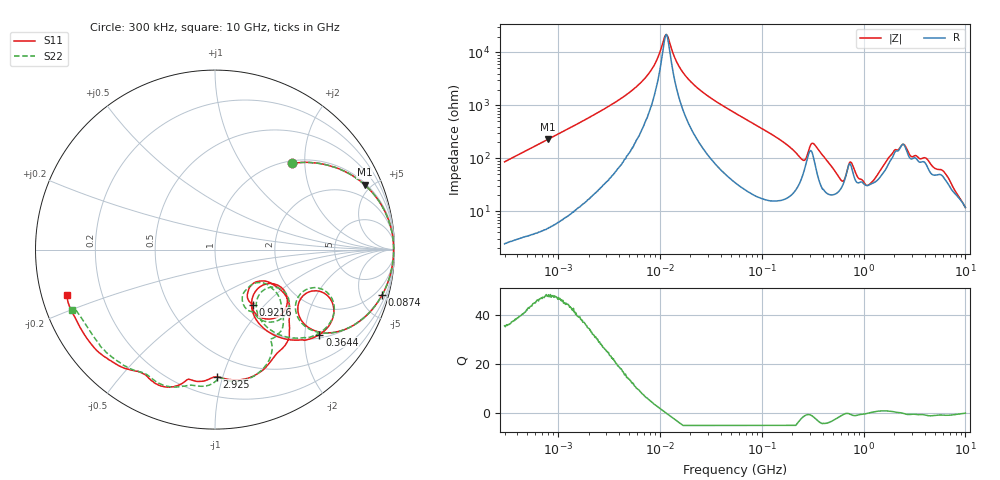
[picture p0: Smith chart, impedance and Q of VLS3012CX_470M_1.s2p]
! S-Parameter Data Generated by TDK Corporation
! Copyright(C) 2019 TDK Corporation.
! All Rights Reserved.
! TDK P/N: VLS3012CX-470M-1 (Inductor)
! Property: L=47uH at 1MHz
! Size(LxWxT): 3x3x1.2mm
! Model Type: s2p (Touchstone File Format Version 1.0)
! Frequency: DC=Yes Start=0.3MHz Stop=10000MHz 802points Log-sweep
! Model Generated on Sep. 23, 2019
! Port Assignments:
!  1 ---@@@--- 2
! Applicable Conditions:
!  Temperature = 25 degC
!  DC Bias Current = 0 A
!  Small Signal Operation
! Terms and conditions regarding TDK Simulation Models
! (1)This simulation model is being provided solely for informational purposes. Please refer to the specifications of the products in terms of detailed characteristics of such products.
! (2)In no event shall TDK Corporation of any of its subsidiaries be liable for any loss or damage arising, directly or indirectly,
!  From any information contained in this simulation model, including, but not limited to loss or damages arising from any inaccuracies, omissions or errors in connection with such information.
! (3)Any and all copyrights on this simulation model are owned by TDK Corporation.
!  Duplication or redistribution of this simulation model without prior written permission from TDK Corporation is prohibited.
! (4)This simulation model is subject to any modification or change without any prior notice.
! (5)Neither TDK Corporation nor any of its subsidiaries shall make any warranty, express or implied,
!  Including but not limited to the correctness, implied warranties of merchantability and fitness for a particular purpose with respect to this simulation models.
! (6)The use of this simulation model shall be deemed to have consented to the terms and conditions hereof.
# Hz S MA R 50
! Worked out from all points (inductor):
!   801 points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, 300 kHz to 10 GHz, reference 50 ohm
!   read as one part in series: L = 45.7 uH near 318.3 kHz
!   highest Q = 47.7 at 796.4 kHz (marker M1), where L = 45.6 uH
!   self-resonance near 11.58 MHz
!   S11 on the Smith chart (normalised r, x): 300 kHz: 1.05, +1.73; 87.4 MHz: 1.00, -7.34; 364.4 MHz: 1.09, -2.37; 921.6 MHz: 1.20, -0.85; 2.925 GHz: 0.34, -0.96; 10 GHz: 0.07, -0.15
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300000  0.6443 48.3  0.7468 -40.1  0.747 -40.1  0.6439 48.3
796418  0.9088 23.4  0.3983 -65.4  0.3985 -65.4  0.9087 23.4
1713600  0.9754 11.3  0.1966 -77.2  0.1965 -77.2  0.9752 11.3
5870124  0.9947 2.4  0.04451 -82.0  0.04446 -82.1  0.9947 2.4
9671944  0.9954 0.4  0.01183 -67.2  0.01185 -67.3  0.9954 0.4
1.174785e7  0.9955 -0.4  0.004634 9.9  0.004639 9.8  0.9954 -0.4
2.036513e7  0.9947 -2.6  0.03616 79.9  0.03618 79.9  0.9946 -2.6
5.477226e7  0.9841 -9.3  0.1363 77.9  0.1364 77.9  0.984 -9.3
8.740098e7  0.9649 -15.2  0.2231 72.2  0.2231 72.2  0.9647 -15.2
2.351426e8  0.6619 -39.9  0.5819 32.6  0.5819 32.6  0.6549 -40.4
3.126428e8  0.7286 -25.3  0.3631 24.7  0.3631 24.7  0.7194 -23.7
3.644326e8  0.7501 -39.2  0.4945 36.4  0.4946 36.4  0.7483 -37.7
5.580434e8  0.4417 -59.5  0.7375 9.5  0.7376 9.5  0.4529 -56.9
6.490631e8  0.3225 -42.9  0.7049 -5.9  0.705 -6.0  0.3505 -41.5
7.318083e8  0.4845 -33.8  0.5321 -5.8  0.5321 -5.8  0.5074 -35.3
9.216398e8  0.3716 -55.6  0.691 -7.4  0.6912 -7.4  0.4122 -58.4
1.276148e9  0.2834 -44.3  0.7169 -30.4  0.717 -30.4  0.2818 -45.1
1.767019e9  0.5152 -36.5  0.4943 -57.4  0.4945 -57.5  0.4843 -40.4
2.477118e9  0.7363 -73.0  0.2645 -49.3  0.2643 -49.3  0.7202 -68.9
2.924554e9  0.7096 -89.0  0.3319 -42.3  0.3318 -42.3  0.7161 -87.0
6.253087e9  0.8345 -128.1  0.2739 -63.2  0.2741 -63.3  0.8211 -128.2
1e10  0.8654 -162.9  0.2293 -89.0  0.2292 -89.1  0.8637 -157.1
